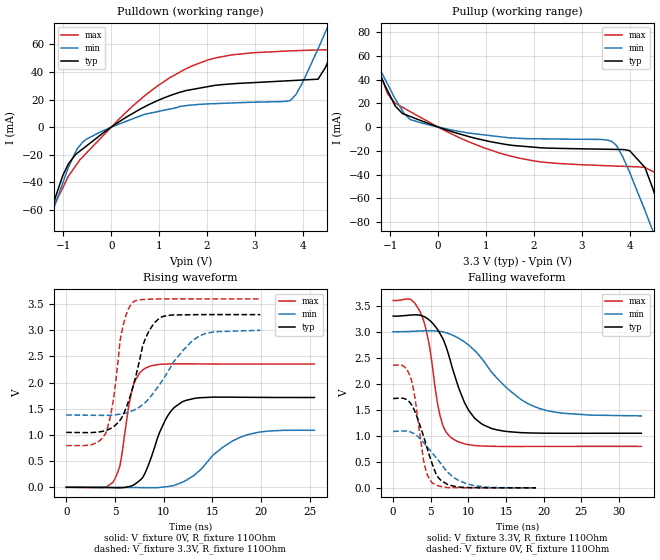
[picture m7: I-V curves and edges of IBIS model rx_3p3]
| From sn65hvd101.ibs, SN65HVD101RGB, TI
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|   rx_3p3 Model
[Model]   rx_3p3
Model_type   Output
Polarity   Inverting
Vmeas = 1.65
Vref = 0
Cref = 2pF
Rref = 200
|   typ   min   max
|   (nom PVT)   (fast PVT)   (slow PVT)
C_comp   2.259e-12   2.233e-12   2.314e-12
| Where nom  PVT is Nominal Process, 3.3V, 45C
|   Fast PVT is Strong Process,  3.6V, -20C
|   Slow PVT is Weak Process,   3V, 125C
[Voltage Range]   3.3   3   3.6
|Junction Temperature
[Temperature Range]   45   125   -20
[Pullup Reference]   3.3   3   3.6
[Pulldown Reference]   0   0   0
[Power Clamp Reference]   3.3   3   3.6
[GND Clamp Reference]   0   0   0
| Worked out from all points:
|   slope of the pulldown table from 0 to 0.495 V, typ, clamps not added: 45.6 ohm
|   slope of the pullup table from 0 to 0.495 V, typ, clamps not added: 78.2 ohm
|   falling waveform, V_fixture 3.3V, R_fixture 110Ohm: 20-80 % time 3.35ns typ, 6.35ns min, 1.92ns max; typ from 3.3 V to 1.05 V
|   rising waveform, V_fixture 0V, R_fixture 110Ohm: 20-80 % time 2.18ns typ, 3.91ns min, 1.23ns max; typ from 0 V to 1.72 V
|   rising waveform, V_fixture 3.3V, R_fixture 110Ohm: 20-80 % time 2.04ns typ, 3.77ns min, 1.25ns max; typ from 1.05 V to 3.3 V
|   falling waveform, V_fixture 0V, R_fixture 110Ohm: 20-80 % time 2.35ns typ, 3.84ns min, 1.41ns max; typ from 1.72 V to 0 V
[Pulldown]
|   Voltage   I(typ)   I(min)   I(max)
-3.3V     -336.2mA   -294.2mA   -406.5mA
-1.307V   -67.3mA    -69.46mA   -71.78mA
-1.013V   -35.16mA   -40.58mA   -44.04mA
-591mV    -15.66mA   -10.72mA   -21.43mA
633.6mV   13.62mA    8.485mA    20.9mA
1.706V    27.41mA    16.09mA    44.69mA
3.744V    33.69mA    19.46mA    55.33mA
4.316V    34.76mA    56.8mA     55.94mA
4.505V    46.02mA    71.77mA    56.1mA
4.838V    76.49mA    98.92mA    57.32mA
5.128V    103.6mA    122.7mA    84.02mA
6.6V      247.8mA    244.6mA    262.6mA
[Pullup]
|   Voltage   I(typ)   I(min)   I(max)
-3.3V     247.5mA    219.5mA    299.6mA
-1.587V   79.74mA    77.92mA    89.06mA
-1.055V   30.51mA    36.05mA    27.88mA
-576mV    8.792mA    6.252mA    12.81mA
1.465V    -14.95mA   -8.993mA   -23.97mA
3.627V    -18.75mA   -12.23mA   -32.73mA
3.996V    -19.85mA   -38.1mA    -33.25mA
4.316V    -34.04mA   -70.18mA   -34.1mA
4.468V    -50.44mA   -86.18mA   -37.08mA
4.727V    -82.02mA   -114.3mA   -47.71mA
4.979V    -113.6mA   -142mA     -81.35mA
6.6V      -336.1mA   -329.5mA   -353mA
[Ramp]
R_load = 110
|   typ   min   max
dV/dt_r   1.02964/2.17412e-09   0.649811/3.85432e-09   1.41302/1.22246e-09
dV/dt_f   1.35067/3.348e-09   0.97122/6.35533e-09   1.6819/1.90699e-09
[Falling Waveform]
V_fixture = 3.3V
V_fixture_min = 3V
V_fixture_max = 3.6V
R_fixture = 110Ohm
|   Time   V(typ)   V(min)   V(max)
0s        3.3V       3V         3.6V
2.25ns    3.319V     3.005V     3.624V
3.58ns    3.317V     3.014V     3.383V
4.77ns    3.228V     3.018V     2.777V
6.24ns    2.963V     3.005V     1.385V
8.22ns    2.144V     2.913V     916.9mV
10.14ns   1.47V      2.731V     827mV
13.29ns   1.132V     2.191V     797.8mV
19.5ns    1.051V     1.521V     796.3mV
33ns      1.049V     1.383V     796.8mV
[Rising Waveform]
V_fixture = 0V
V_fixture_min = 0V
V_fixture_max = 0V
R_fixture = 110Ohm
|   Time   V(typ)   V(min)   V(max)
0s        1.83nV     14.46nV    1.334nV
4.78ns    -7.656mV   -918uV     94.72mV
5.51ns    -10.41mV   -1.84mV    413.6mV
6.36ns    10.02mV    -3.214mV   1.492V
6.85ns    39.6mV     -4.156mV   1.923V
8.17ns    306.2mV    -7.182mV   2.282V
10.15ns   1.281V     7.671mV    2.355V
12.04ns   1.646V     108.1mV    2.359V
17.83ns   1.72V      955.1mV    2.355V
25.46ns   1.716V     1.09V      2.355V
[Rising Waveform]
V_fixture = 3.3V
V_fixture_min = 3V
V_fixture_max = 3.6V
R_fixture = 110Ohm
|   Time   V(typ)   V(min)   V(max)
0s        1.049V     1.381V     796.8mV
4.04ns    1.085V     1.375V     1.025V
4.78ns    1.149V     1.381V     1.608V
5.68ns    1.328V     1.403V     2.959V
6.21ns    1.55V      1.425V     3.331V
6.98ns    2.013V     1.477V     3.555V
8.08ns    2.823V     1.618V     3.59V
9.86ns    3.261V     2.042V     3.6V
13.56ns   3.299V     2.88V      3.6V
19.9ns    3.3V       3V         3.6V
[Falling Waveform]
V_fixture = 0V
V_fixture_min = 0V
V_fixture_max = 0V
R_fixture = 110Ohm
|   Time   V(typ)   V(min)   V(max)
0s        1.716V     1.083V     2.355V
1.36ns    1.719V     1.094V     2.342V
2.32ns    1.623V     1.073V     2.119V
2.93ns    1.455V     1.026V     1.7V
4.09ns    970.6mV    863.2mV    498mV
4.54ns    755.2mV    786.3mV    254.4mV
5.21ns    454.9mV    669mV      93.63mV
6.43ns    133.7mV    449.6mV    22.38mV
9.95ns    4.816mV    70.53mV    1.169mV
19ns      1.794nV    14.47nV    1.337nV
